|Texas Instruments Incorporated
|tmux7209, 4 Data Lane 2:1 MIPI Switch (10-Channel, 2:1 Analog Switch)
[IBIS Ver]   4.1
[File name]   tmux7209.ibs
[Date]   03/09/21
[File Rev]   1.0
[Source]
| Texas Instruments Incorporated.
| ASC-INT-MPD
| 12500 TI Blvd
| Dallas, TX - 75243
[Notes]   Revision History:
| Rev 1.0: 03/09/21
| - Initial version of the model
| - Model generated from simulations in SPECTRE
| - C_comp although listed in numerical order of value are
|   obtained from varying PVT conditions. For PVT conditions for
|   each specific value refer the buffer description under
|   respective [Model]. IBIS model user is responsible for using
|   appropriate C_comp to simulate for Signal Integrity.
[Disclaimer]
| This model is designed as an aid for customers of Texas Instruments.
| TI and its licensors and suppliers make no warranties, either expressed
| or implied, with respect to this  model, including the warranties of
| merchantability or fitness for a particular purpose. The model is
| provided solely on an "as is" basis. The entire risk as to its quality
| and performance is with the customer.
| This model is subject to change without notice. Texas Instruments
| Incorporated is not responsible for updating this model.
[Copyright]
(C) Copyright 2021 Texas Instruments Incorporated.All rights reserved.
|  Component TMUX7209PW 16-pin - PW package
|  Part # TMUX7209PW
[Component]   TMUX7209PW
[Manufacturer]  TI
[Package]
|   typ   min   max
R_pkg   0.05   NA   NA
L_pkg   1.0nH   NA   NA
C_pkg   0.2pF   NA   NA
[Pin]   signal_name   model_name
   1   A0   inbuf
   2   EN   inbuf
   3   VSS   POWER
   4   S1A   sterm
   5   S2A   sterm
   6   S3A   sterm
   7   S4A   sterm
   8   DA   dterm
   9   DB   dterm
   10   S4B   sterm
   11   S3B   sterm
   12   S2B   sterm
   13   S1B   sterm
   14   VDD   POWER
   15   GND   GND
   16   A1   inbuf
[Series Switch Groups]
On 1 /
On 2 /
On 3 /
On 4 /
Off 1 2 3 4 /
[Series Pin Mapping]  pin_2 model_name function_table_group
|   4   8   switch_dual_5   1
|  13   9   switch_dual_5   1
|   5   8   switch_dual_5   2
|  12   9   switch_dual_5   2
|   6   8   switch_dual_5   3
|  11   9   switch_dual_5   3
|   7   8   switch_dual_5   4
|  10   9   switch_dual_5   4
   4   8   switch_dual_20   1
  13   9   switch_dual_20   1
   5   8   switch_dual_20   2
  12   9   switch_dual_20   2
   6   8   switch_dual_20   3
  11   9   switch_dual_20   3
   7   8   switch_dual_20   4
  10   9   switch_dual_20   4
|   4   8   switch_dual_15   1
|  13   9   switch_dual_15   1
|   5   8   switch_dual_15   2
|  12   9   switch_dual_15   2
|   6   8   switch_dual_15   3
|  11   9   switch_dual_15   3
|   7   8   switch_dual_15   4
|  10   9   switch_dual_15   4
|   4   8   switch_36   1
|  13   9   switch_36   1
|   5   8   switch_36   2
|  12   9   switch_36   2
|   6   8   switch_36   3
|  11   9   switch_36   3
|   7   8   switch_36   4
|  10   9   switch_36   4
|   4   8   switch_44   1
|  13   9   switch_44   1
|   5   8   switch_44   2
|  12   9   switch_44   2
|   6   8   switch_44   3
|  11   9   switch_44   3
|   7   8   switch_44   4
|  10   9   switch_44   4
|   4   8   switch_12   1
|  13   9   switch_12   1
|   5   8   switch_12   2
|  12   9   switch_12   2
|   6   8   switch_12   3
|  11   9   switch_12   3
|   7   8   switch_12   4
|  10   9   switch_12   4
|  Component TMUX7209RRP 16-pin - RRP package
|  Part # TMUX7209RRP
[Component]   TMUX7209RRP
[Manufacturer]  TI
[Package]
|   typ   min   max
R_pkg   0.05   NA   NA
L_pkg   1.0nH   NA   NA
C_pkg   0.2pF   NA   NA
[Pin]   signal_name   model_name
   1   VSS   POWER
   2   S1A   sterm
   3   S2A   sterm
   4   S3A   sterm
   5   S4A   sterm
   6   DA   dterm
   7   DB   dterm
   8   S4B   sterm
   9   S3B   sterm
   10   S2B   sterm
   11   S1B   sterm
   12   VDD   POWER
   13   GND   GND
   14   A1   inbuf
   15   A0   inbuf
   16   EN   inbuf
[Series Switch Groups]
On 1 /
On 2 /
On 3 /
On 4 /
Off 1 2 3 4 /
[Series Pin Mapping]  pin_2 model_name function_table_group
   2   6   switch_dual_5   1
  11   7   switch_dual_5   1
   3   6   switch_dual_5   2
  10   7   switch_dual_5   2
   4   6   switch_dual_5   3
   9   7   switch_dual_5   3
   5   6   switch_dual_5   4
   8   7   switch_dual_5   4
|   2   6   switch_dual_20   1
|  11   7   switch_dual_20   1
|   3   6   switch_dual_20   2
|  10   7   switch_dual_20   2
|   4   6   switch_dual_20   3
|   9   7   switch_dual_20   3
|   5   6   switch_dual_20   4
|   8   7   switch_dual_20   4
|   2   6   switch_dual_15   1
|  11   7   switch_dual_15   1
|   3   6   switch_dual_15   2
|  10   7   switch_dual_15   2
|   4   6   switch_dual_15   3
|   9   7   switch_dual_15   3
|   5   6   switch_dual_15   4
|   8   7   switch_dual_15   4
|   2   6   switch_36   1
|  11   7   switch_36   1
|   3   6   switch_36   2
|  10   7   switch_36   2
|   4   6   switch_36   3
|   9   7   switch_36   3
|   5   6   switch_36   4
|   8   7   switch_36   4
|   2   6   switch_44   1
|  11   7   switch_44   1
|   3   6   switch_44   2
|  10   7   switch_44   2
|   4   6   switch_44   3
|   9   7   switch_44   3
|   5   6   switch_44   4
|   8   7   switch_44   4
|   2   6   switch_12   1
|  11   7   switch_12   1
|   3   6   switch_12   2
|  10   7   switch_12   2
|   4   6   switch_12   3
|   9   7   switch_12   3
|   5   6   switch_12   4
|   8   7   switch_12   4
[Model Selector] dterm
dterm_dual_5 Use for operation at +/-5V
dterm_dual_20 Use for operation at +/-20V
dterm_dual_15 Use for operation at +/-15V
dterm_36 Use for operation at 36V
dterm_44 Use for operation at 44V
dterm_12 Use for operation at 12V
[Model Selector] sterm
sterm_dual_5 Use for operation at +/-5V
sterm_dual_20 Use for operation at +/-20V
sterm_dual_15 Use for operation at +/-15V
sterm_36 Use for operation at 36V
sterm_44 Use for operation at 44V
sterm_12 Use for operation at 12V
[Model Selector] inbuf
inbuf_dual_5 Use for operation at +/-5V
inbuf_dual_20 Use for operation at +/-20V
inbuf_dual_15 Use for operation at +/-15V
inbuf_36 Use for operation at 36V
inbuf_44 Use for operation at 44V
inbuf_12 Use for operation at 12V
| switch_dual_5
[Model]   switch_dual_5
Model_type   Series_switch
|   typ   min   max
C_comp   1.598234e-11   NA   NA
[Voltage Range]   0   -5   5
[Temperature Range]   27   NA   NA
[On]
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[Off]
|   typ   min   max
[R Series]   10G   NA   NA
| switch_dual_20
[Model]   switch_dual_20
Model_type   Series_switch
|   typ   min   max
C_comp   4.014581e-11   NA   NA
[Voltage Range]   0   -20   20
[Temperature Range]   27   NA   NA
[On]
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[Off]
|   typ   min   max
[R Series]   10G   NA   NA
| switch_dual_15
[Model]   switch_dual_15
Model_type   Series_switch
|   typ   min   max
C_comp   2.533030e-11   NA   NA
[Voltage Range]   0   -15   15
[Temperature Range]   27   NA   NA
[On]
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[Off]
|   typ   min   max
[R Series]   10G   NA   NA
| switch_36
[Model]   switch_36
Model_type   Series_switch
|   typ   min   max
C_comp   4.014581e-11   NA   NA
[Voltage Range]   36   0   36
[Temperature Range]   27   NA   NA
[On]
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[Off]
|   typ   min   max
[R Series]   10G   NA   NA
| switch_44
[Model]   switch_44
Model_type   Series_switch
|   typ   min   max
C_comp   4.014581e-11   NA   NA
[Voltage Range]   44   0   44
[Temperature Range]   27   NA   NA
[On]
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[Off]
|   typ   min   max
[R Series]   10G   NA   NA
| switch_12
[Model]   switch_12
Model_type   Series_switch
|   typ   min   max
C_comp   1.598234e-11   NA   NA
[Voltage Range]   12   0   12
[Temperature Range]   27   NA   NA
[On]
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[Off]
|   typ   min   max
[R Series]   10G   NA   NA
| Models and submodels in the file (24): dterm_dual_5 (Terminator), dterm_dual_20 (Terminator), dterm_dual_15 (Terminator), dterm_36 (Terminator), dterm_44 (Terminator), dterm_12 (Terminator), switch_dual_5 (Series_switch), switch_dual_20 (Series_switch), switch_dual_15 (Series_switch), switch_36 (Series_switch), switch_44 (Series_switch), switch_12 (Series_switch), sterm_dual_5 (Terminator), sterm_dual_20 (Terminator), sterm_dual_15 (Terminator), sterm_36 (Terminator), sterm_44 (Terminator), sterm_12 (Terminator), inbuf_dual_5 (Input), inbuf_dual_20 (Input), inbuf_dual_15 (Input), inbuf_36 (Input), inbuf_44 (Input), inbuf_12 (Input)
